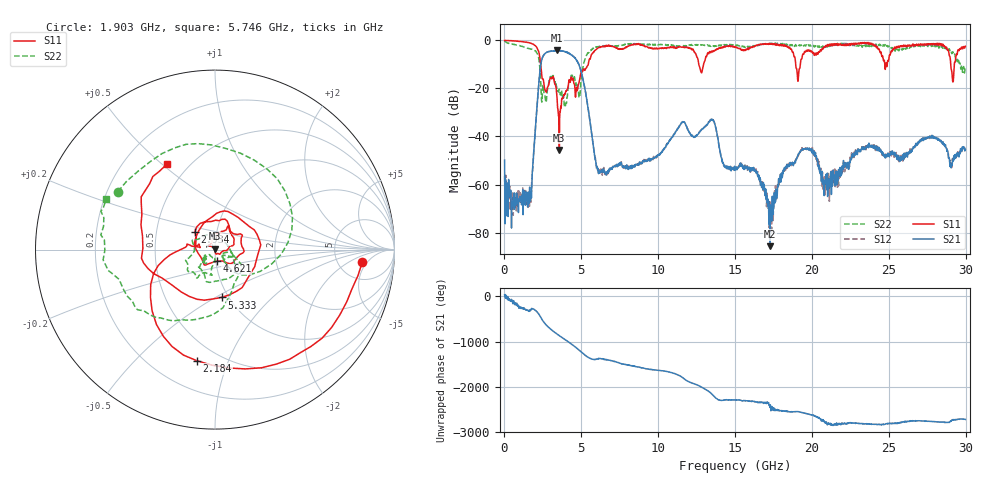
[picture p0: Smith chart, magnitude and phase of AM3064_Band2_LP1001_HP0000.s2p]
# Hz S DB R 50.0
!freq dBS11 angS11 dBS21 angS21 dBS12 angS12 dBS22 angS22
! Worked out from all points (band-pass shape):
!   1600 points, 10 MHz to 29.98 GHz, reference 50 ohm
!   highest |S21| = -4.12 dB at 3.403 GHz (marker M1); lowest = -85.7 dB at 17.27 GHz (marker M2)
!   |S21| within 3 dB of the highest: 2.472 GHz to 4.558 GHz (2.086 GHz wide, 59.4 % of centre)
!   lowest |S11| = -45.6 dB at 3.571 GHz (marker M3), VSWR 1.01, Z = 49.7 + j0.458 ohm
!   |S11| at or under -10 dB: 2.358 GHz to 5.451 GHz (3.092 GHz wide, 79.2 % of centre); 12.64 GHz to 12.95 GHz (308.6 MHz wide, 2.41 % of centre); 18.94 GHz to 19.25 GHz (304.7 MHz wide, 1.6 % of centre)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
!   |S22| runs from -27.8 to -0.3 dB; largest |S21 - S12| = 0.019
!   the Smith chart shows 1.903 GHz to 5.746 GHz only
!   S11 on the Smith chart (normalised r, x): 1.903 GHz: 8.68, -3.78; 2.184 GHz: 0.38, -0.78; 2.934 GHz: 0.79, +0.16; 4.621 GHz: 1.01, -0.13; 5.333 GHz: 0.93, -0.53; 5.746 GHz: 0.38, +0.52
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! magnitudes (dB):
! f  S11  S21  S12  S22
! 10 MHz  0.0  -49.8  -56.5  -0.3
! 1.566 GHz  -0.9  -63.4  -64.5  -3.3
! 1.903 GHz  -1.7  -46.5  -46.7  -4.0
! 2.184 GHz  -4.0  -21.9  -22.0  -6.2
! 2.54 GHz  -16.8  -6.3  -6.2  -19.6
! 2.934 GHz  -16.6  -4.7  -4.6  -15.9
! 3.403 GHz  -22.6  -4.1  -4.3  -19.8
! 3.571 GHz  -45.6  -4.2  -4.3  -20.3
! 4.621 GHz  -23.6  -7.5  -7.6  -18.9
! 5.015 GHz  -13.0  -13.5  -13.5  -14.8
! 5.333 GHz  -11.4  -23.8  -23.7  -6.3
! 5.746 GHz  -5.3  -42.3  -42.4  -3.5
! 6.214 GHz  -3.0  -55.2  -54.7  -2.4
! 10 GHz  -3.4  -47.8  -47.1  -1.8
! 13.49 GHz  -4.6  -32.9  -32.8  -2.3
! 15 GHz  -2.6  -53.9  -53.3  -1.8
! 16.35 GHz  -2.3  -55.1  -54.4  -2.5
! 17.27 GHz  -1.4  -85.7  -75.2  -1.2
! 19.99 GHz  -4.6  -45.2  -45.6  -2.0
! 20.8 GHz  -2.7  -64.6  -56.8  -2.6
! 25 GHz  -8.0  -47.6  -47.4  -2.3
! 29.98 GHz  -2.4  -45.5  -45.5  -10.8
